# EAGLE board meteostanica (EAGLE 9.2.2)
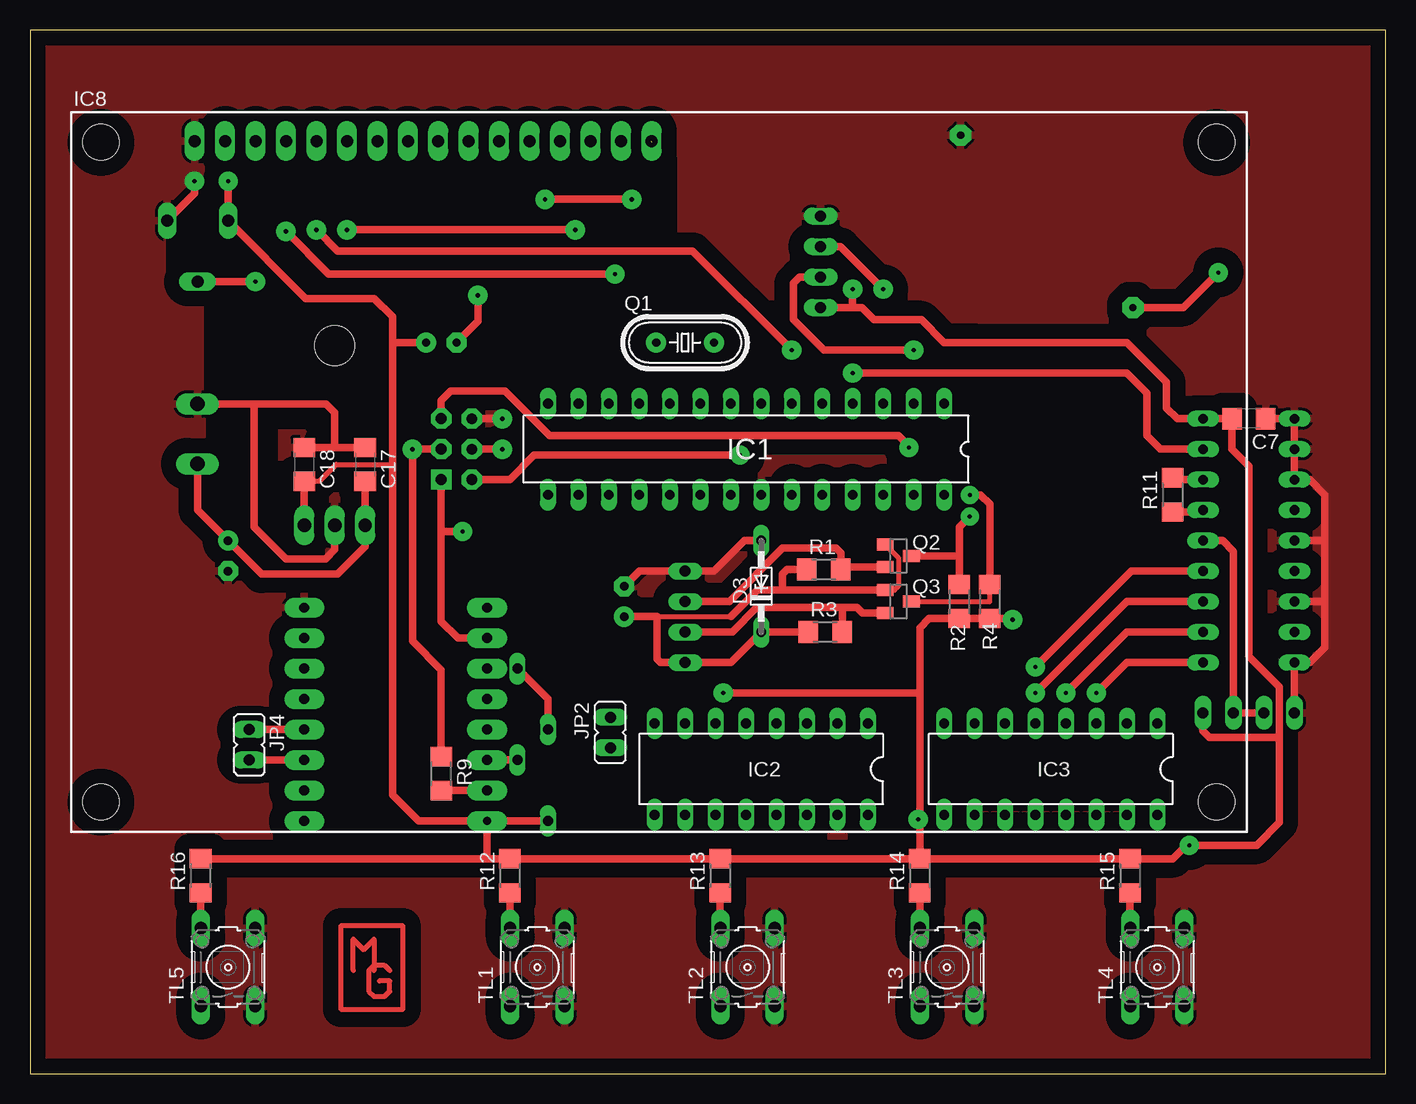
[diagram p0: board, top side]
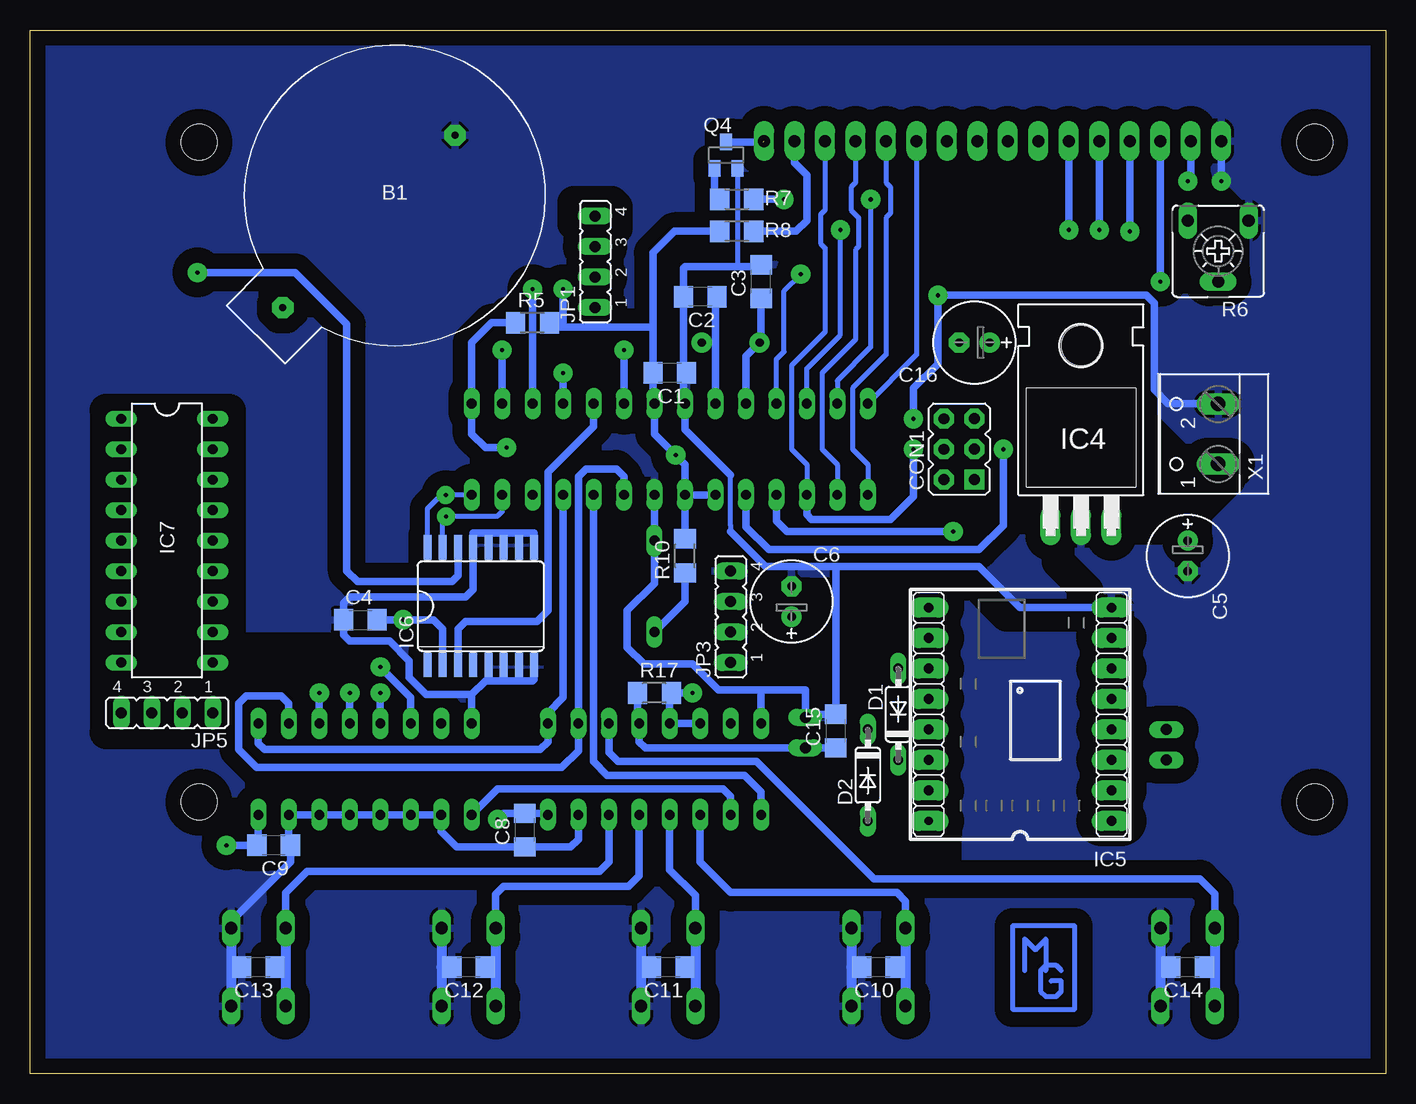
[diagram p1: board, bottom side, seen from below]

Size 113.02 x 87.02 mm. Coordinates in mm from the lower left corner, seen from the top.
Outline: 0,0 113,0 113.02,87.02 0,87 0,0
Copper layers (1*16): Top 0.035mm / dielectric 1.5mm / Bottom 0.035mm
Design rules "default": minimum track width 6mil, minimum drill 0.35mm, track to track 6mil, track to pad 6mil, pad to pad 6mil, via to via 6mil, smd to smd 6mil, copper to edge 40mil, drill to drill 6mil, minimum pad ring 10mil, minimum via ring 8mil, stop-mask expansion 4mil, vias tented up to drill 0mil, thermal gap 10mil
bKeepout: 1 lines
tRestrict: 69 lines
bRestrict: area 96.4,28.4 to 106.7,55.3; 122 lines

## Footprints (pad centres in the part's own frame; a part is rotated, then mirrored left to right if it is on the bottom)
CR2032 = drill 0.6 pad 1.778 octagon: + 0,0; - -20.32,0
C1206 = smd 1.6 x 1.8: 1 -1.4,0; 2 1.4,0
E2,5-7 = drill 0.7 pad 1.676: + -1.27,0 | drill 0.7 pad 1.676 octagon: - 1.27,0
CON-ISP6 = drill 0.914 pad 1.676 square: 1 -2.54,-1.27 | drill 0.9 pad 1.676 octagon: 2 -2.54,1.27; 4 0,1.27; 6 2.54,1.27 | drill 0.914 pad 1.676 octagon: 3 0,-1.27; 5 2.54,-1.27
DO35-7 = drill 0.813 long: A 3.81,0; C -3.81,0
DO34Z7 = drill 0.813 long: A 3.81,0; C -3.81,0
DIL28-3 = drill 0.813 long: 1 -16.51,-3.81; 2 -13.97,-3.81; 3 -11.43,-3.81; 4 -8.89,-3.81; 5 -6.35,-3.81; 6 -3.81,-3.81; 7 -1.27,-3.81; 8 1.27,-3.81; 9 3.81,-3.81; 10 6.35,-3.81; 11 8.89,-3.81; 12 11.43,-3.81; 13 13.97,-3.81; 14 16.51,-3.81; 15 16.51,3.81; 16 13.97,3.81; 17 11.43,3.81; 18 8.89,3.81; 19 6.35,3.81; 20 3.81,3.81; 21 1.27,3.81; 22 -1.27,3.81; 23 -3.81,3.81; 24 -6.35,3.81; 25 -8.89,3.81; 26 -11.43,3.81; 27 -13.97,3.81; 28 -16.51,3.81
DIL16 = drill 0.813 long: 1 -8.89,-3.81; 2 -6.35,-3.81; 3 -3.81,-3.81; 4 -1.27,-3.81; 5 1.27,-3.81; 6 3.81,-3.81; 7 6.35,-3.81; 8 8.89,-3.81; 9 8.89,3.81; 10 6.35,3.81; 11 3.81,3.81; 12 1.27,3.81; 13 -1.27,3.81; 14 -3.81,3.81; 15 -6.35,3.81; 16 -8.89,3.81
TO220H = drill 1.118 long: 1 -2.54,-10.16; 2 0,-10.16; 3 2.54,-10.16 | hole 3.302: 0,4.826
WT588D = drill 0.813 pad 1.676 long: 1 -8.89,-7.62; 2 -6.35,-7.62; 3 -3.81,-7.62; 4 -1.27,-7.62; 5 1.27,-7.62; 6 3.81,-7.62; 7 6.35,-7.62; 8 8.89,-7.62; 9 8.89,7.62; 10 6.35,7.62; 11 3.81,7.62; 12 1.27,7.62; 13 -1.27,7.62; 14 -3.81,7.62; 15 -6.35,7.62 | drill 0.7 pad 1.676 long: 16 -8.89,7.62
SO16L = smd 0.66 x 2.032: 1 -4.445,-4.902; 2 -3.175,-4.902; 3 -1.905,-4.902; 4 -0.635,-4.902; 5 0.635,-4.902; 6 1.905,-4.902; 7 3.175,-4.902; 8 4.445,-4.902; 9 4.445,4.902; 10 3.175,4.902; 11 1.905,4.902; 12 0.635,4.902; 13 -0.635,4.902; 14 -1.905,4.902; 15 -3.175,4.902; 16 -4.445,4.902
DIL18 = drill 0.813 long: 1 -10.16,-3.81; 2 -7.62,-3.81; 3 -5.08,-3.81; 4 -2.54,-3.81; 5 0,-3.81; 6 2.54,-3.81; 7 5.08,-3.81; 8 7.62,-3.81; 9 10.16,-3.81; 10 10.16,3.81; 11 7.62,3.81; 12 5.08,3.81; 13 2.54,3.81; 14 0,3.81; 15 -2.54,3.81; 16 -5.08,3.81; 17 -7.62,3.81; 18 -10.16,3.81
LCD20X4_HOLES = drill 1 pad 1.676 long: 1 10.3,-2.4; 2 12.84,-2.4; 3 15.38,-2.4; 4 17.92,-2.4; 5 20.46,-2.4; 6 23,-2.4; 7 25.54,-2.4; 8 28.08,-2.4; 9 30.62,-2.4; 10 33.16,-2.4; 11 35.7,-2.4; 12 38.24,-2.4; 13 40.78,-2.4; 14 43.32,-2.4; 15 45.86,-2.4; 16 48.4,-2.4 | hole 3: 2.5,-2.5; 95.5,-2.5; 2.5,-57.5; 95.5,-57.5
JP4 = drill 0.914 long: 1 -3.81,0; 2 -1.27,0; 3 1.27,0; 4 3.81,0
JP1 = drill 0.914 long: 1 0,-1.27; 2 0,1.27
HC49/S = drill 0.7 pad 1.676: 1 -2.413,0; 2 2.413,0
SOT23 = smd 1 x 1.4: 1 -0.95,-1.1; 2 0.95,-1.1; 3 0,1.1
R1206 = smd 1.6 x 1.803: 1 -1.422,0; 2 1.422,0
CA6V = drill 1.016 long: A -2.54,-2.54; E 2.54,-2.54; S 0,2.54
B3F-10XX = drill 1.016 long: 1 -3.251,2.261; 2 3.251,2.261; 3 -3.251,-2.261; 4 3.251,-2.261
W237-102 = drill 1.194 long: 1 -2.5,-1.27; 2 2.5,-1.27

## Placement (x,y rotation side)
B1  CR2032  [CR2032]  91.95,63.88 225 bottom
C1  100n  [C1206]  59.69,58.42 180 bottom
C2  22p  [C1206]  57.15,64.77 180 bottom
C3  22p  [C1206]  52.07,66.04 90 bottom
C4  100n  [C1206]  85.47,37.85 0 bottom
C5  47u  [E2,5-7]  16.51,43.18 270 bottom
C6  47u  [E2,5-7]  49.53,39.37 90 bottom
C7  100n  [C1206]  101.6,54.61 180 top
C8  100n  [C1206]  71.75,20.32 90 bottom
C9  100n  [C1206]  92.71,19.05 180 bottom
C10  100n  [C1206]  42.29,8.89 180 bottom
C11  100n  [C1206]  59.82,8.89 180 bottom
C12  100n  [C1206]  76.45,8.89 180 bottom
C13  100n  [C1206]  93.98,8.89 180 bottom
C14  100n  [C1206]  16.51,8.89 180 bottom
C15  100n  [C1206]  45.85,28.57 90 bottom
C16  47u  [E2,5-7]  34.29,60.96 180 bottom
C17  100n  [C1206]  27.94,50.8 270 top
C18  100n  [C1206]  22.86,50.8 270 top
CON1  CON-ISP6  [CON-ISP6]  35.56,52.07 90 bottom
D1  1N4148  [DO35-7]  40.64,29.97 90 bottom
D2  1N4148  [DO35-7]  43.18,24.89 270 bottom
D3  3V3  [DO34Z7]  60.96,40.64 90 top
IC1  MEGA328-P  [DIL28-3]  59.69,52.07 180 top
IC2  74165N  [DIL16]  60.96,25.4 180 top
IC3  74165N  [DIL16]  85.09,25.4 180 top
IC4  7805T  [TO220H]  25.4,55.88 0 bottom
IC5  WT588D  [WT588D]  30.48,29.97 90 bottom
IC6  DS3231  [SO16L]  75.44,38.99 0 bottom
IC7  HT12D  [DIL18]  101.6,44.45 270 bottom
IC8  LCD20X4  [LCD20X4_HOLES]  3.42,80.16 0 top
JP1  REČ  [JP4]  65.91,67.69 90 bottom
JP2  [JP1]  48.39,28.45 180 top
JP3  SHTC3  [JP4]  54.61,38.1 90 bottom
JP4  AUDIO  [JP1]  18.29,27.43 180 top
JP5  RECEIVER  [JP4]  101.6,30.1 180 bottom
Q1  8MHz  [HC49/S]  54.61,60.96 0 top
Q2  BSS138  [SOT23]  72.39,43.18 270 top
Q3  BSS138  [SOT23]  72.39,39.37 270 top
Q4  BSS138  [SOT23]  54.99,76.58 0 bottom
R1  10k  [R1206]  66.17,42.04 0 top
R2  10k  [R1206]  77.47,39.37 90 top
R3  10k  [R1206]  66.29,36.83 0 top
R4  10k  [R1206]  80.01,39.37 90 top
R5  10k  [R1206]  71.12,62.61 0 bottom
R6  10k  [CA6V]  13.97,68.58 180 bottom
R7  560  [R1206]  54.1,70.23 0 bottom
R8  10k  [R1206]  54.1,72.9 180 bottom
R9  10k  [R1206]  34.29,25.02 270 top
R10  560  [R1206]  58.42,43.18 270 bottom
R11  100k  [R1206]  95.25,48.26 90 top
R12  10k  [R1206]  40.01,16.51 90 top
R13  10k  [R1206]  57.53,16.51 90 top
R14  10k  [R1206]  74.17,16.51 90 top
R15  10k  [R1206]  91.69,16.51 90 top
R16  10k  [R1206]  14.22,16.51 90 top
R17  10k  [R1206]  60.96,31.75 0 bottom
TL1  [B3F-10XX]  42.29,8.89 90 top
TL2  [B3F-10XX]  59.82,8.89 90 top
TL3  [B3F-10XX]  76.45,8.89 90 top
TL4  [B3F-10XX]  93.98,8.89 90 top
TL5  [B3F-10XX]  16.51,8.89 90 top
U$1  [#MG3-VECTOR]  25.4,5.08 0 top
U$2  [#MG3-VECTOR]  31.62,5.08 0 bottom
X1  POWER  [W237-102]  15.24,53.34 90 bottom

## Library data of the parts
B1 CON1 IC5-IC8 Q2-Q4 U$1 U$2 = #Matej
C1-C18 R1-R5 R7-R17 = rcl
D1-D3 = diode
IC1 = atmel; OC_FARNELL: unknown; OC_NEWARK: unknown
IC2 IC3 = 74xx-eu
IC4 = linear
JP1-JP5 = jumper
Q1 = crystal; OC_FARNELL: 1667008; OC_NEWARK: unknown
R6 = pot
TL1-TL5 = switch-omron; MPN: B3F-1000; OC_FARNELL: 176432; OC_NEWARK: 36M3542
X1 = con-wago-500; MPN: 237-102; OC_FARNELL: unknown; OC_NEWARK: 70K9898

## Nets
+3V3: C6.+ D3.C JP3.1 Q2.1 Q3.1 R1.1 R3.1 R10.2
+5V: C1.2 C4.2 C7.2 C8.2 C9.2 C16.+ C18.2 CON1.2 D2.A IC1.7 IC1.20 IC1.21 IC2.5 IC2.6 IC2.16 IC3.16 IC4.3 IC5.16 IC6.2 IC7.18 IC8.2 JP1.1 JP5.1 R2.1 R4.1 R5.2 R6.E R7.1 R10.1 R12.2 R13.2 R14.2 R15.2 R16.2 R17.2
GND: B1.- C1.1 C2.2 C3.2 C4.1 C5.- C6.- C7.1 C8.1 C9.1 C10.2 C11.2 C12.2 C13.2 C14.2 C15.2 C16.- C17.1 C18.1 CON1.6 D3.A IC1.8 IC1.22 IC2.8 IC2.15 IC3.8 IC3.10 IC3.11 IC3.12 IC3.13 IC3.14 IC3.15 IC4.2 IC5.8 IC6.5 IC6.6 IC6.7 IC6.8 IC6.9 IC6.10 IC6.11 IC6.12 IC6.13 IC7.1 IC7.2 IC7.3 IC7.5 IC7.7 IC7.9 IC8.1 JP1.4 JP2.1 JP3.4 JP5.4 Q4.2 R6.A TL1.3 TL1.4 TL2.3 TL2.4 TL3.3 TL3.4 TL4.3 TL4.4 TL5.3 TL5.4 X1.2
INT0: IC1.4 IC7.17
LCD_D4: IC1.14 IC8.11
LCD_D5: IC1.15 IC8.12
LCD_D6: IC1.16 IC8.13
LCD_E: IC1.12 IC8.6
LCD_LIGHT: IC1.13 R8.1
LCD_R/W: IC1.6 IC8.5
LCD_RS: IC1.11 IC8.4
MISO: CON1.1 IC1.18 IC5.10
MOSI: CON1.4 IC1.17 IC8.14
N$1: IC2.10 IC3.9
N$2: IC7.16 R11.2
N$3: C3.1 IC1.10 Q1.1
N$4: IC7.15 R11.1
N$5: C2.1 IC1.9 Q1.2
N$6: C14.1 IC2.3 R16.1 TL5.1 TL5.2
N$7: IC8.3 R6.S
N$8: IC8.15 R7.2
N$9: IC8.16 Q4.3
N$10: Q4.1 R8.2
N$11: D1.A D2.C
N$12: D1.C IC5.14
N$13: IC5.15 R9.2
N$14: IC1.5 IC6.3
N$15: B1.+ IC6.14
N$16: C13.1 IC2.14 R15.1 TL4.1 TL4.2
N$17: C12.1 IC2.13 R14.1 TL3.1 TL3.2
N$18: C11.1 IC2.12 R13.1 TL2.1 TL2.2
N$19: C10.1 IC2.11 R12.1 TL1.1 TL1.2
N$20: IC7.14 JP5.2 JP5.3
N$22: C5.+ C17.2 IC4.1 X1.1
N$23: IC5.4 JP4.1
N$24: IC5.3 JP4.2
N$32: C15.1 IC2.4 JP2.2 R17.1
RESET: CON1.5 IC1.1 R5.1
RX: IC1.2 JP1.2
RX_D8: IC3.3 IC7.10
RX_D9: IC3.4 IC7.11
RX_D10: IC3.5 IC7.12
RX_D11: IC3.6 IC7.13
SCK: CON1.3 IC1.19 R9.1
SCL_3V3: JP3.2 Q3.2 R3.2
SCL_5V: IC1.28 IC6.16 Q3.3 R4.2
SDA_3V3: JP3.3 Q2.2 R1.2
SDA_5V: IC1.27 IC6.15 Q2.3 R2.2
SHF_CLK: IC1.23 IC2.2 IC3.2
SHF_DATA: IC1.24 IC2.9
SHF_SH/LD: IC1.25 IC2.1 IC3.1
TX: IC1.3 JP1.3

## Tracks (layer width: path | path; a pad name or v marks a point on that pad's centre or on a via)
+3V3
  Top 0.406: 52.27,38.12 58.45,38.12 | Q2.1 72.39,43.03 72.39,40.64 72.07,40.32 Q3.1
  Top 0.61: R3.1 64.14,36.83 D3.C 58.42,34.29 JP3.1 52.58,34.29 52.27,34.59 52.27,38.12 49.55,38.12 C6.+ | R1.1 63.12,42.04 62.74,41.66 62.74,40.32 | Q3.1 62.74,40.32 | 58.45,38.12 60.64,40.32 62.74,40.32
  Bottom 0.61: R10.2 58.42,39.37 D3.C
+5V  (via drill 0.35 pad 1.6)
  Top 0.406: C18.2 24.13,49.4 25.53,50.8 30.23,50.8
  Top 0.61: R14.2 R15.2 95.28,17.93 96.39,19.05 v96.65,19.05 102.25,19.05 104.14,20.94 104.14,28.06 | R14.2 R13.2 R12.2 38.1,17.93 | 38.1,17.93 27.94,17.93 R16.2 | v74.04,21.21 74.17,21.08 | 74.17,21.08 R14.2 | v16.51,74.42 R6.E 22.99,64.64 28.7,64.64 30.23,63.12 30.23,60.96 | IC5.16 32.38,21.08 30.23,23.24 30.23,50.8 30.23,60.96 | CON1.2 40.01,49.53 42.04,51.56 57.02,51.56 59.17,51.56 v59.18,51.58 | v81.92,37.85 81.81,37.95 R4.1 R2.1 74.93,37.95 74.17,37.19 74.17,31.75 | 74.17,31.75 74.17,21.08 | IC5.16 D2.A | IC5.16 38.1,17.93 | C16.+ 30.23,60.96 | C18.2 IC4.3 | v57.78,31.75 74.17,31.75 | 68.58,63.88 69.34,63.88 70.36,62.87 74.3,62.87 76.2,60.96 78.74,60.96 91.44,60.96 94.74,57.66 94.74,55.5 95.63,54.61 IC7.18 C7.2 100.2,52.07 101.6,50.67 101.6,34.8 104.14,32.26 104.14,28.45 104.14,28.06 | 68.58,63.88 JP1.1 | 68.58,63.88 v68.58,65.41 | JP5.1 97.79,28.59 98.32,28.06 104.14,28.06
  Bottom 0.61: IC2.16 69.98,21.72 C8.2 73.53,21.72 73.66,21.59 v74.04,21.21 | IC6.2 78.61,37.08 79.38,37.85 v81.92,37.85 | v81.92,37.85 82.04,37.85 v81.92,37.85 | IC3.16 93.98,19.18 C9.2 v96.65,19.05 | C4.2 v81.92,37.85 | 16.26,74.67 v16.51,74.42 16.26,74.67 | R7.1 59.31,70.23 61.09,68.45 61.09,62.23 | 61.09,62.23 C1.2 61.09,56.01 IC1.7 60.96,53.34 v59.19,51.57 | IC1.20 IC1.21 | IC1.21 58.42,50.8 v59.19,51.57 | v59.18,51.58 v59.19,51.57 | IC1.21 R10.1 | IC2.6 IC2.5 59.69,31.6 R17.2 v57.78,31.75 | R5.2 69.32,62.23 68.58,62.23 | 68.58,62.23 61.09,62.23 | v68.58,65.41 68.58,62.23 | IC8.2 16.26,74.67
GND  (via drill 0.35 pad 1.6)
  Top 0.61: C7.1 IC7.1 IC7.2 IC7.3 106.68,49.53 107.95,48.26 107.95,44.45 | 107.95,44.45 107.95,39.37 | 107.95,39.37 107.95,35.56 106.68,34.29 IC7.9 JP5.4 | IC7.7 107.95,39.37 | IC7.5 107.95,44.45 | v13.72,74.42 13.72,73.41 R6.A | C16.- 37.34,62.74 v37.34,64.9 | X1.2 18.67,55.84 | 18.67,55.84 24.68,55.84 25.4,55.12 25.4,52.32 25.28,52.2 | C17.1 25.28,52.2 | 25.28,52.2 25.27,52.2 C18.1 | IC4.2 25.4,43.69 24.64,42.93 21.34,42.93 18.67,45.59 18.67,55.84 | D3.A 59.56,44.45 57.02,41.91 JP3.4 50.8,41.91 C6.- | CON1.6 v39.37,54.61
  Bottom 0.406: Q4.2 54.04,67.37 54.1,67.31 | 54.61,45.21 54.61,45.72 54.61,49.91
  Bottom 0.61: IC2.15 67.31,19.56 67.95,18.92 C8.1 77.47,18.92 78.74,20.19 IC3.10 IC3.11 IC3.12 IC3.13 IC3.14 IC3.15 91.44,19.18 C9.1 91.31,17.66 96.24,12.72 TL4.4 | 74.8,45.09 76.07,45.09 IC6.13 76.07,40.39 76.71,39.75 86.36,39.75 86.87,39.24 C4.1 86.87,36.58 86.36,36.07 83.06,36.07 81.41,34.42 81.41,33.02 80.01,31.62 76.2,31.62 | 74.8,45.09 73.53,45.09 | 73.53,45.09 72.14,45.09 | 72.14,45.09 70.99,45.09 IC6.9 | IC6.10 72.26,44.96 72.14,45.09 | IC6.11 73.53,45.09 | IC6.12 74.8,45.09 | 74.8,32.77 IC6.5 | IC6.8 70.99,32.89 71.12,32.77 72.39,32.77 | 72.39,32.77 73.53,32.77 | 73.53,32.77 74.8,32.77 | IC6.6 73.53,32.77 | IC6.7 72.26,32.89 72.39,32.77 | 76.2,31.62 IC3.8 | 76.2,31.62 75.06,32.77 74.8,32.77 | C3.2 52.2,67.31 54.1,67.31 58.42,67.31 58.55,67.18 C2.2 58.55,58.42 | 58.55,58.42 58.55,56.01 IC1.8 58.42,53.7 58.4,53.7 54.61,49.91 | C1.1 58.55,58.42 | v13.72,74.42 13.72,77.73 IC8.1 | IC1.22 D3.A 60.96,40.89 63.25,38.61 63.25,35.56 61.85,34.16 57.78,34.16 55.63,32 52.07,32 | 52.07,32 48.39,32 JP2.1 48.13,29.98 C15.2 45.85,42.29 | IC2.8 52.07,32 | IC5.8 30.48,38.86 33.91,42.29 45.85,42.29 | 54.61,45.21 51.69,42.29 46.99,42.29 45.85,42.29 | v39.37,54.61 39.37,57.15 37.34,59.18 v37.34,64.9 19.94,64.9 19.3,64.26 19.3,57.02 18.16,55.88 14.01,55.88 X1.2
  Bottom 0.813: TL5.4 18.77,8.89 | 18.77,8.89 TL5.3 | C14.2 18.77,8.89 | TL1.4 44.55,8.89 | 44.55,8.89 TL1.3 | C10.2 44.55,8.89 | TL2.4 62.08,8.89 | 62.08,8.89 TL2.3 | C11.2 62.08,8.89 | TL3.4 78.72,8.89 | 78.72,8.89 TL3.3 | C12.2 78.72,8.89 | TL4.4 96.24,8.89 | 96.24,8.89 TL4.3 | C13.2 96.24,8.89
  pour Top (isolate 1.27): 0,0 113.03,0 113.03,87.63 0,87.63
  pour Bottom (isolate 1.27): 0,0 113.03,0 113.03,87.63 0,87.63
INT0  (via drill 0.35 pad 1.6)
  Top 0.61: IC7.17 95.89,52.07 94.23,52.07 93.09,53.21 93.09,56.77 91.44,58.42 89.53,58.42 v68.58,58.42
  Bottom 0.61: v68.58,58.42 IC1.4
LCD_D4
  Bottom 0.406: IC1.14 39.37,59.69 39.12,59.94 IC8.11
LCD_D5
  Bottom 0.406: IC1.15 43.18,50.8 44.45,52.07 44.45,57.15 41.66,59.94 41.66,71.37 41.27,71.75 41.27,73.91 41.66,74.3 IC8.12
LCD_D6
  Bottom 0.406: IC1.16 45.72,50.8 46.99,52.07 46.99,58.42 44.2,61.21 44.2,68.7 43.94,68.96 43.94,71.37 44.58,72.01 44.58,73.91 44.2,74.3 IC8.13
LCD_E  (via drill 0.35 pad 1.6)
  Top 0.61: v45.47,70.36 v26.42,70.36
  Bottom 0.406: IC1.12 48.26,58.8 45.47,61.59 v45.47,70.36
  Bottom 0.61: v26.42,70.36 26.42,77.73 IC8.6
LCD_LIGHT  (via drill 0.35 pad 1.6)
  Top 0.61: v50.16,72.9 v42.94,72.9 | v42.94,72.9 42.93,72.9 v42.94,72.9
  Bottom 0.406: v42.94,72.9 42.94,60.56 45.72,57.78 IC1.13
  Bottom 0.61: R8.1 v50.16,72.9
LCD_R/W  (via drill 0.35 pad 1.6)
  Top 0.61: v63.5,60.33 55.24,68.58 25.65,68.58 v23.88,70.36
  Bottom 0.61: IC1.6 v63.5,60.33 | v23.88,70.36 23.88,77.73 IC8.5
LCD_RS  (via drill 0.35 pad 1.6)
  Top 0.61: v48.77,66.67 24.89,66.67 v21.34,70.23
  Bottom 0.406: IC1.11 50.8,59.56 50.16,60.2 50.16,65.28 v48.77,66.67
  Bottom 0.61: v21.34,70.23 21.34,77.73 IC8.4
MISO  (via drill 0.35 pad 1.6)
  Top 0.61: 34.29,45.21 34.29,37.72 35.69,36.32 IC5.10 | 34.29,45.21 CON1.1 | v36.07,45.21 34.29,45.21
  Bottom 0.61: v36.07,45.21 49.91,45.21 50.8,46.1 IC1.18
MOSI  (via drill 0.35 pad 1.6)
  Top 0.61: v39.37,52.07 CON1.4
  Bottom 0.406: IC1.17 48.26,50.8 49.53,52.07 49.53,59.05 46.74,61.84 46.74,68.84 47.12,69.22 47.12,71.63 46.74,72.01 IC8.14
  Bottom 0.61: IC1.17 48.26,46.61 47.88,46.23 41.27,46.23 39.37,48.13 v39.37,52.07
N$1
  Bottom 0.61: IC2.10 54.61,23.11 55.24,23.75 74.04,23.75 IC3.9
N$2
  Top 0.61: R11.2 95.4,49.53 IC7.16
N$3
  Bottom 0.61: C3.1 52.07,61.09 Q1.1 53.34,59.82 IC1.10
N$4
  Top 0.61: R11.1 97.64,46.84 IC7.15
N$5
  Bottom 0.61: IC1.9 55.88,60.96 | 55.88,60.96 55.88,64.64 C2.1 | Q1.2 55.88,60.96
N$6
  Top 0.61: R16.1 14.22,12.17 TL5.2
  Bottom 0.61: TL5.2 14.25,15.01 15.49,16.26 42.67,16.26 52.45,26.04 64.01,26.04 64.77,26.8 IC2.3
  Bottom 0.813: TL5.2 14.25,8.89 | 14.25,8.89 TL5.1 | C14.1 14.25,8.89
N$7  (via drill 0.35 pad 1.6)
  Top 0.61: R6.S v18.8,66.04
  Bottom 0.61: v18.8,66.04 | IC8.3 v18.8,66.04
N$8
  Bottom 0.61: R7.2 49.15,70.23 48.26,71.12 48.26,74.93 49.28,75.95 IC8.15
N$9  (1 unrouted)
  Bottom 0.61: 51.87,77.68 Q4.3
N$10
  Bottom 0.61: Q4.1 55.94,73.31 R8.2
N$11
  Top 0.61: D1.A 43.18,31.24 D2.C
N$12
  Top 0.61: D1.C IC5.14
N$13
  Top 0.61: R9.2 34.31,23.62 IC5.15
N$14
  Bottom 0.61: IC6.3 77.34,37.08 76.71,37.72 70.74,37.72 69.85,38.61 69.85,50.16 66.04,53.98 IC1.5
N$15  (via drill 0.35 pad 1.6)
  Top 0.61: B1.+ 96.14,63.88 v99.06,66.8
  Bottom 0.61: IC6.14 77.34,41.53 77.85,41.02 85.72,41.02 86.61,41.91 86.61,62.48 90.93,66.8 v99.06,66.8
N$16
  Top 0.61: R15.1 91.69,12.17 TL4.2
  Bottom 0.61: IC2.14 64.77,17.65 65.53,16.89 89.92,16.89 91.72,15.09 TL4.2
  Bottom 0.813: TL4.2 91.72,8.89 | 91.72,8.89 TL4.1 | C13.1 91.72,8.89
N$17
  Top 0.61: R14.1 74.17,12.17 TL3.2
  Bottom 0.61: IC2.13 62.23,16.51 63.12,15.62 73.53,15.62 74.19,14.96 TL3.2
  Bottom 0.813: TL3.2 74.19,8.89 | 74.19,8.89 TL3.1 | C12.1 74.19,8.89
N$18
  Top 0.61: R13.1 57.53,12.17 TL2.2
  Bottom 0.61: IC2.12 59.69,17.02 57.53,14.86 57.53,12.17 TL2.2
  Bottom 0.813: TL2.2 57.56,8.89 | 57.56,8.89 TL2.1 | C11.1 57.56,8.89
N$19
  Top 0.61: R12.1 40.01,12.17 TL1.2
  Bottom 0.61: TL1.2 40.03,14.38 40.77,15.11 54.61,15.11 57.15,17.65 IC2.11
  Bottom 0.813: TL1.2 40.03,8.89 | 40.03,8.89 TL1.1 | C10.1 40.03,8.89
N$20
  Top 0.61: JP5.3 JP5.2 100.33,43.56 99.44,44.45 IC7.14
N$22
  Top 0.61: X1.1 13.97,46.99 C5.+ 19.3,41.66 25.65,41.66 27.94,43.94 IC4.1 C17.2
N$23
  Top 0.61: JP4.1 IC5.4
N$24
  Top 0.61: JP4.2 IC5.3
N$32
  Bottom 0.61: R17.1 62.38,29.36 IC2.4 62.23,27.69 61.72,27.18 JP2.2 C15.1
RESET  (via drill 0.35 pad 1.6)
  Top 0.61: CON1.5 34.29,56.13 35.05,56.9 39.62,56.9 43.31,53.21 72.39,53.21 73.28,52.32 v73.28,52.2
  Bottom 0.61: v73.28,52.2 75.06,52.2 76.2,53.34 IC1.1 76.2,60.96 74.55,62.61 R5.1
RX  (via drill 0.35 pad 1.6)
  Top 0.61: v73.66,60.33 66.17,60.33 63.63,62.87 63.63,65.91 64.14,66.42 JP1.2
  Bottom 0.61: v73.66,60.33 IC1.2
RX_D8  (via drill 0.35 pad 1.6)
  Top 0.61: IC7.10 91.44,34.29 v88.9,31.75
  Bottom 0.61: IC3.3 v88.9,31.75
RX_D9  (via drill 0.35 pad 1.6)
  Top 0.61: IC7.11 91.44,36.83 v86.36,31.75
  Bottom 0.61: v86.36,31.75 IC3.4
RX_D10  (via drill 0.35 pad 1.6)
  Top 0.61: v83.82,31.75 91.44,39.37 IC7.12
  Bottom 0.61: IC3.5 v83.82,31.75
RX_D11  (via drill 0.35 pad 1.6)
  Top 0.61: IC7.13 91.82,41.91 v83.82,33.91
  Bottom 0.61: v83.82,33.91 81.28,31.37 IC3.6
SCK  (via drill 0.35 pad 1.6)
  Top 0.61: CON1.3 v31.88,52.07 31.88,36.07 34.29,33.66 R9.1
  Bottom 0.61: IC1.19 53.34,45.59 51.44,43.69 33.91,43.69 31.88,45.72 v31.88,52.07
SCL_3V3
  Top 0.61: JP3.2 58.55,36.83 60.58,38.86 67.69,38.86 | Q3.2 69.39,38.42 68.94,38.86 67.69,38.86 | R3.2 67.72,38.84 67.69,38.86
SCL_5V  (via drill 0.35 pad 1.5)
  Top 0.406: Q3.3 80.01,39.37 R4.2
  Top 0.61: R4.2 80.01,47.5 79.25,48.26 v78.36,48.26
  Bottom 0.406: IC1.28 v78.36,48.26 78.74,48.26 79.88,47.12 IC6.16
SDA_3V3
  Top 0.61: Q2.2 67.78,42.23 R1.2 67.59,43.41 67.18,43.81 62.74,43.81 58.29,39.37 JP3.3
SDA_5V  (via drill 0.35 pad 1.5)
  Top 0.61: R2.2 77.47,43.18 | 77.47,43.18 77.47,45.59 v78.34,46.46 | Q2.3 77.47,43.18
  Bottom 0.406: IC1.27 73.66,46.86 74.04,46.48 78.32,46.48 v78.34,46.46 78.61,46.19 IC6.15
SHF_CLK
  Bottom 0.61: IC1.23 63.5,49.78 64.14,50.42 66.67,50.42 67.31,49.78 IC2.2 67.31,26.92 68.71,25.53 94.11,25.53 95.63,27.05 95.63,30.86 95,31.5 92.08,31.5 91.44,30.86 IC3.2
SHF_DATA
  Bottom 0.61: IC2.9 52.07,23.5 53.47,24.89 64.9,24.89 66.04,26.04 IC1.24
SHF_SH/LD
  Bottom 0.61: IC1.25 68.58,31.37 69.85,30.1 IC2.1 69.85,27.69 70.48,27.05 93.47,27.05 93.98,27.56 IC3.1
TX  (via drill 0.35 pad 1.6)
  Top 0.61: v71.12,65.41 67.56,68.96 JP1.3
  Bottom 0.61: IC1.3 v71.12,65.41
